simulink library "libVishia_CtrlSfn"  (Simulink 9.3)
settings: Solver=VariableStepAuto  StartTime=0.0  StopTime=10.0  RelTol=1e-3
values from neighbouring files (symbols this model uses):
  Tinit = 0.001    [TestOrthOsc_init.m]    (also in Test_PIDctrl_init.m)
  Tstep = 0.000050    (= 5e-05)    [TestOrthOsc_init.m]    (also in Test_PIDctrl_init.m = 0.0001)
undefined symbols (not defined in the file or in its folder): avgSteps, incrAvgSteps, P_WaveData_FB, P_WaveMng_FB, P_WaveMngIx_FB, src2genBus, stepA_WaveMngIx_FB, stepSimulink_AvgWave_FB, stepSimulink_WaveData_FB, stepSimulink_WaveMng_FB, u1, u2, void, work1, y1
libraries: lib_WaveMng x20, $bdroot x8, Lib_FunctionBlocks x4, lib_Conv x2

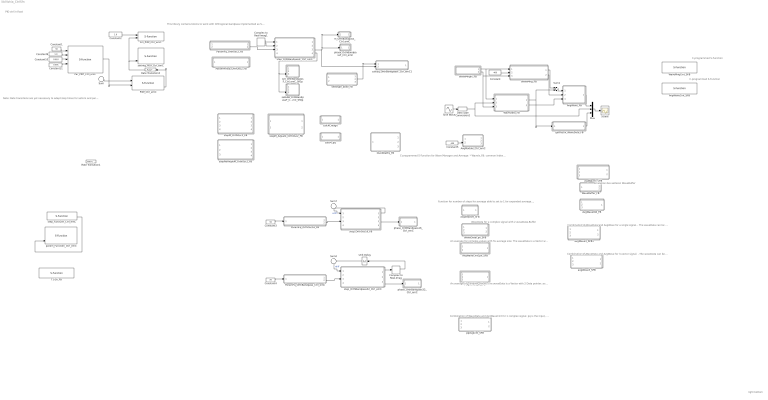
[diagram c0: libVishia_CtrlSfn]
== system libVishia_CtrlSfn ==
  note: Note: Rate transitions are yet necessary to adapt step times for setLim and param FBlock. The Limitation and parametrization may be occure in another step time. Note "step time" is the "sample time" in Simulink. "step" means more the control step.
  note: right bottom
  note: PID ctrl in float
  note: This library contains blocks to work with Orthogonal bandpass implemented as S-Function
  note: C-programmed S-Function
  note: C-programmed S-Function
  note: An average for complex values. The waveData is a Vector with 2 Data pointer. avg is a complex output.
  note: Function for number of steps for average able to set to 1 for expanded average. Parameter avgSteps
  note: C-programmed S-Function for Wave Manager and Average: * WaveIx_FB: common Index for one Buffer size. * WaveMng_FB: common manager for one average period but maybe more as one signal for averaging. * WaveData_FB; Buffer for data, for one signal value, but maybe for more as one average * AvgWave_FB: average for one signal and period. The connections ..._FB are references (ObjectOriented). The connections step... are only used to determine the calculation order.
  note: Combination of WaveData and AvgWaveCint for 1 complex signal. pq is the input, avg is the output. The waveData can be used for other accesses. It is a vector o2 2 pointer.
  note: An average for complex values with fix average size. The waveData is a Vector with 2 Data pointer. avg is a complex output.
  note: WaveData for a complex signal with 2 waveData-Buffer
  note: Emulation des aelteren WaveBuffer
  note: Combination of WaveData and AvgWave for a single signal. . The waveData can be used for other accesses. It is a pointer.
  note: Combination of WaveData and AvgWave for 3-vector signal. . The waveData can be used for other accesses. It is a vector o2 3 pointer.
  AvgModule_Ctrl_emC : Subsystem
  AvgWaveCintCpx_SFB : Subsystem
  AvgWaveCint_SFB : S-Function  LoadFcn=defWaveMngPtr  FunctionName=AvgWaveCint_SFB  SFunctionDeploymentMode=off  EnableBusSupport=off
  AvgWaveCpx_SFB : Subsystem
  AvgWaveOld_FB : Subsystem
  AvgWave_FB : Subsystem
  Complex to Real-Imag : ComplexToRealImag
  Complex to Real-Imag1 : ComplexToRealImag
  Constant : Constant  Value=400  OutDataTypeStr=single
  Constant1 : Constant  Value=50  OutDataTypeStr=single  SampleTime=-1
  Constant10 : Constant  Value=0.010  OutDataTypeStr=single  SampleTime=-1
  Constant11 : Constant  Value=0.001  OutDataTypeStr=single  SampleTime=-1
  Constant2 : Constant  Value=1.0  OutDataTypeStr=single  SampleTime=-1
  Constant3 : Constant  Value=50  OutDataTypeStr=single
  Constant4 : Constant  Value=50  OutDataTypeStr=single
  Constant5 : Constant  Value=400  OutDataTypeStr=single
  Constant9 : Constant  Value=1.0  OutDataTypeStr=single  SampleTime=-1
  Data Type Conversion2 : DataTypeConversion  OutDataTypeStr=single
  Mux : Mux  Inputs=3
  OscillDetFq_FB : Subsystem
  PIDf_Ctrl_emC : S-Function  FunctionName=step_PIDf_Ctrl_emC_SfH  Parameters=Tstep  SFunctionDeploymentMode=off  EnableBusSupport=off
  Par_PIDf_Ctrl_emC : S-Function  FunctionName=set_Par_PIDf_Ctrl_emC_SfH  Parameters=Tctrl yMax openLoop Tparam  SFunctionDeploymentMode=off  EnableBusSupport=off
  ParamFq_OrthBandpass_Ctrl_emC : Subsystem
  ParamFq_OrthOsc16_FB : Subsystem
  ParamFq_OrthOsc2_FB : Subsystem
  ParamPeriod_OrthOsc2_FB : Subsystem
  Rate Transition1 : RateTransition  OutPortSampleTimeOpt=Inherit  OutPortSampleTime=Tinit
  Rate Transition3 : RateTransition  OutPortSampleTimeOpt=Inherit  OutPortSampleTime=1.0
  Scope : Scope
  Sine Wave : Sin  Amplitude=4  Frequency=10.02*pi  SampleTime=Tstep
  Sum : Sum  Inputs=|+-
  Sum1 : Sum
  Sum2 : Sum  Inputs=+|-
  Sum7 : Sum  Inputs=+|-
  T1i16_FB : S-Function  FunctionName=stepY_T1i_Ctrl_emC_SfH  Parameters=Ts Tstep  SFunctionDeploymentMode=off  EnableBusSupport=off
  Unit Delay : UnitDelay  SampleTime=-1  HasFrameUpgradeWarning=on
  WaveBuffer_FB : Subsystem
  WaveDataCpx_SFB : Subsystem
  WaveData_FB : Subsystem
  WaveMngCint_SFB : S-Function  FunctionName=WaveMngCint_SFB  SFunctionDeploymentMode=off  EnableBusSupport=off
  WaveMngIx_FB : Subsystem
  WaveMng_FB : Subsystem
  avgStepSet_SFB : Subsystem
  avgWave3_CFB : Subsystem
  avgWave3_SFB : Subsystem
  avgWave3_SFB1 : Subsystem
  calcM_magn : Subsystem  TreatAsAtomicUnit=on
  calcM_pq : Subsystem  TreatAsAtomicUnit=on
  calcdq_OrthBandpassF_Ctrl_emC1 : Subsystem
  getPastIx_WaveData_FB : Subsystem
  lim_PIDf_Ctrl_emC : S-Function  FunctionName=setLim_PIDf_Ctrl_emC_SfOp  SFunctionDeploymentMode=off  EnableBusSupport=off
  m_OrthBandpass_Ctrl_emC : Subsystem
  param_FuncGen_Ctrl_emC : S-Function  FunctionName=param_FuncGen_Ctrl_emC_SfOp  SFunctionDeploymentMode=off  EnableBusSupport=off
  phase_OrthBandpass16_Ctrl_emC : Subsystem
  phase_OrthBandpass32_Ctrl_emC : Subsystem
  phase_OrthBandpassF_Ctrl_emC : Subsystem
  pqAvgCint_SFB : Subsystem
  setAngle_abwf_FB : Subsystem
  setIntg_PIDf_Ctrl_emC : S-Function  FunctionName=setIntg_PIDf_Ctrl_emC_SfOp  SFunctionDeploymentMode=off  EnableBusSupport=off
  set_OrthBandpassF_Ctrl_emC_SfOp : Subsystem
  setkAB_OrthBandpassF_Ctrl_emC_SfOp : Subsystem
  stepM_Adjustk_OrthOsc2_FB : Subsystem  TreatAsAtomicUnit=on
  stepM_OrthOsc2_FB : Subsystem  TreatAsAtomicUnit=on
  stepNoAngleM_OrthOsc2_FB : Subsystem  TreatAsAtomicUnit=on
  step_FuncGen_Ctrl_emC : S-Function  FunctionName=step_FuncGen_Ctrl_emC_SfH  Parameters=Tstep  SFunctionDeploymentMode=off  EnableBusSupport=off
  step_OrthBandpass32_Ctrl_emC : Subsystem
  step_OrthBandpassF_Ctrl_emC : Subsystem  LoadFcn=src2genBus.lib_OrthOsc_genBus();
  step_OrthOsc16_FB : Subsystem
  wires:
  Sum/1 -> PIDf_Ctrl_emC/1
  ? -> Sum/1  "w"
  ? -> Sum/2  "x"
  PIDf_Ctrl_emC/3 -> Rate Transition3/1
  Sum1/1 -> AvgWave_FB/1(In1)
  Data Type Conversion2/1 -> WaveData_FB/2(In3), Mux/2
  WaveMngIx_FB/2(Out1) -> WaveMng_FB/3(In2), WaveData_FB/3(In2)
  Constant/1 -> WaveMng_FB/2(In3)
  Sine Wave/1 -> Data Type Conversion2/1
  WaveData_FB/1(Out2) -> getPastIx_WaveData_FB/1(In2), Sum1/2
  WaveMng_FB/1(Out2) -> Sum1/1
  getPastIx_WaveData_FB/1(Out2) -> Mux/3
  WaveMng_FB/2(Out1) -> AvgWave_FB/2(In2)
  Mux/1 -> Scope/1
  WaveMngIx_FB/1(Out2) -> WaveData_FB/1(In1), WaveMng_FB/1(In1)
  WaveData_FB/2(Out1) -> AvgWave_FB/3(In4)
  AvgWave_FB/1(Out2) -> Mux/1
  Constant1/1 -> Par_PIDf_Ctrl_emC/1
  Constant10/1 -> Par_PIDf_Ctrl_emC/3
  Constant9/1 -> Par_PIDf_Ctrl_emC/2
  Constant11/1 -> Par_PIDf_Ctrl_emC/4
  Constant2/1 -> lim_PIDf_Ctrl_emC/1
  Par_PIDf_Ctrl_emC/1 -> PIDf_Ctrl_emC/2
  Rate Transition3/1 -> lim_PIDf_Ctrl_emC/2, setIntg_PIDf_Ctrl_emC/4
  ParamFq_OrthOsc16_FB/2(Out2) -> step_OrthOsc16_FB/3(In1)
  Sum7/1 -> step_OrthOsc16_FB/1(In4)  "xdiff"
  step_OrthOsc16_FB/1(Out3) -> Sum7/2
  ? -> Sum7/1
  Constant3/1 -> ParamFq_OrthOsc16_FB/1(In1)
  ? -> ?
  step_FuncGen_Ctrl_emC/2 -> param_FuncGen_Ctrl_emC/4
  ParamFq_OrthBandpass_Ctrl_emC/2(Out2) -> step_OrthBandpass32_Ctrl_emC/3(In1)
  Constant4/1 -> ParamFq_OrthBandpass_Ctrl_emC/1(In1)
  Sum2/1 -> step_OrthBandpass32_Ctrl_emC/1(In4)  "xdiff"
  Complex to Real-Imag/1 -> Unit Delay/1
  ? -> Sum2/1
  step_OrthBandpass32_Ctrl_emC/1(Out4) -> Complex to Real-Imag/1
  Unit Delay/1 -> Sum2/2
  Constant5/1 -> AvgModule_Ctrl_emC/2(In3)
  step_OrthBandpass32_Ctrl_emC/3(Out1) -> phase_OrthBandpass32_Ctrl_emC/1(In1)
  Complex to Real-Imag1/1 -> step_OrthBandpassF_Ctrl_emC/1(In4)
  Complex to Real-Imag1/2 -> step_OrthBandpassF_Ctrl_emC/2(In5)
  ParamFq_OrthOsc2_FB/2(Out2) -> step_OrthBandpassF_Ctrl_emC/3(In1)
  step_OrthBandpassF_Ctrl_emC/3(thiz_OrthOsc2_FB1) -> phase_OrthBandpassF_Ctrl_emC/1(In3), m_OrthBandpass_Ctrl_emC/1(In3), calcdq_OrthBandpassF_Ctrl_emC1/2(In3)
  step_OrthBandpassF_Ctrl_emC/4(thiz_OrthOsc2_FB) -> setkAB_OrthBandpassF_Ctrl_emC_SfOp/3(In3), set_OrthBandpassF_Ctrl_emC_SfOp/3(In3)
  setAngle_abwf_FB/2(thiz_Angle_abwmf_FB2) -> calcdq_OrthBandpassF_Ctrl_emC1/1(In1)
  step_OrthOsc16_FB/3(Out2) -> phase_OrthBandpass16_Ctrl_emC/1(In1)

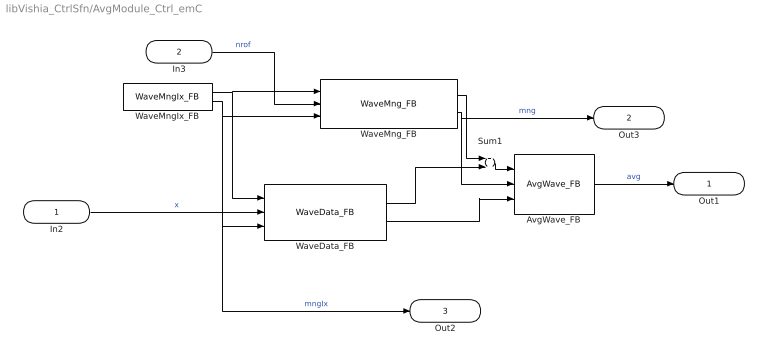
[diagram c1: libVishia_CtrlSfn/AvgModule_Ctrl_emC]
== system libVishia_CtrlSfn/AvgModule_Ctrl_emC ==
  In2 : Inport  OutDataTypeStr=single  PortDimensions=1
  In3 : Inport  Port=2  OutDataTypeStr=single  PortDimensions=1
  AvgWave_FB : $bdroot/AvgWave_FB  identObj=1
  Sum1 : Sum
  WaveData_FB : $bdroot/WaveData_FB  identObj=1  size=1024
  WaveMngIx_FB : $bdroot/WaveMngIx_FB  identObj=1  size=1024  Tstep=Tstep
  WaveMng_FB : $bdroot/WaveMng_FB  identObj=1
  Out1 : Outport  OutDataTypeStr=single  PortDimensions=1
  Out3 : Outport  Port=2  OutDataTypeStr=uint32  PortDimensions=1
  Out2 : Outport  Port=3  OutDataTypeStr=uint32  PortDimensions=1
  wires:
  WaveData_FB/1 -> Sum1/2
  WaveData_FB/2 -> AvgWave_FB/3
  WaveMngIx_FB/1 -> WaveData_FB/1, WaveMng_FB/1
  In3/1 -> WaveMng_FB/2  "nrof"
  In2/1 -> WaveData_FB/2  "x"
  WaveMng_FB/2 -> AvgWave_FB/2, Out3/1  "mng"
  Sum1/1 -> AvgWave_FB/1
  WaveMng_FB/1 -> Sum1/1
  WaveMngIx_FB/2 -> WaveMng_FB/3, Out2/1, WaveData_FB/3  "mngIx"
  AvgWave_FB/1 -> Out1/1  "avg"

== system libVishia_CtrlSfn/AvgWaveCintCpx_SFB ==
  In1 : Inport
  In5 : Inport  Port=2  OutDataTypeStr=P_WaveData_FB  PortDimensions=2
  AvgWaveCint_SFB : lib_WaveMng/AvgWaveCint_SFB  SFunctionSpec=stepSimulink_AvgWave_FB(void* work1, P_WaveMng_FB u1, P_WaveData_FB u2, single y1[1])  ShowSpec=off
  AvgWaveCint_SFB1 : lib_WaveMng/AvgWaveCint_SFB  SFunctionSpec=stepSimulink_AvgWave_FB(void* work1, P_WaveMng_FB u1, P_WaveData_FB u2, single y1[1])  ShowSpec=off
  Demux : Demux  Outputs=2
  Real-Imag to Complex2 : RealImagToComplex
  Out2 : Outport
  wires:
  In1/1 -> AvgWaveCint_SFB1/1, AvgWaveCint_SFB/1  "waveMngCiint"
  AvgWaveCint_SFB1/1 -> Real-Imag to Complex2/2
  Demux/1 -> AvgWaveCint_SFB/2  "waveD_xUApq[0]"
  AvgWaveCint_SFB/1 -> Real-Imag to Complex2/1
  In5/1 -> Demux/1  "waveData"
  Real-Imag to Complex2/1 -> Out2/1  "avg"
  Demux/2 -> AvgWaveCint_SFB1/2  "waveD_xUApq[1]"

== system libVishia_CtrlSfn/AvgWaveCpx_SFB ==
  In2 : Inport
  In1 : Inport  Port=2  OutDataTypeStr=uint32
  In5 : Inport  Port=3  OutDataTypeStr=uint32  PortDimensions=2
  AvgWave_FB : $bdroot/AvgWave_FB  identObj=0
  AvgWave_FB1 : $bdroot/AvgWave_FB  identObj=0
  Demux : Demux  Outputs=2
  Real-Imag to Complex2 : RealImagToComplex
  Out2 : Outport  OutDataTypeStr=single
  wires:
  Demux/2 -> AvgWave_FB1/3  "waveD_xUApq[1]"
  Real-Imag to Complex2/1 -> Out2/1  "avg"
  In5/1 -> Demux/1  "waveData"
  AvgWave_FB/1 -> Real-Imag to Complex2/1
  Demux/1 -> AvgWave_FB/3  "waveD_xUApq[0]"
  AvgWave_FB1/1 -> Real-Imag to Complex2/2
  In1/1 -> AvgWave_FB1/2, AvgWave_FB/2  "waveMng"
  In2/1 -> AvgWave_FB1/1, AvgWave_FB/1  "step"

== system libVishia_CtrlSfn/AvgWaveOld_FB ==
  In6 : Inport  OutDataTypeStr=P_WaveMngIx_FB
  In2 : Inport  Port=2  OutDataTypeStr=P_WaveData_FB
  In1 : Inport  Port=3  OutDataTypeStr=P_WaveMngIx_FB  PortDimensions=1
  AvgWave_SFB : lib_WaveMng/AvgWave_SFB  SFunctionSpec=stepSimulink_AvgWave_FB(void* work1, P_WaveMng_FB u1, P_WaveData_FB u2, single y1[1])  ShowSpec=off
  WaveMng_SFB : lib_WaveMng/WaveMng_SFB  SFunctionSpec=stepSimulink_WaveMng_FB(void* work1, P_WaveMngIx_FB u1, single u2, P_WaveMng_FB y1[1])  ShowSpec=off
  Out1 : Outport  OutDataTypeStr=single
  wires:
  WaveMng_SFB/1 -> AvgWave_SFB/1
  In6/1 -> WaveMng_SFB/1  "waveIxP"
  In1/1 -> WaveMng_SFB/2  "N"
  In2/1 -> AvgWave_SFB/2  "waveDataP"
  AvgWave_SFB/1 -> Out1/1  "Y"

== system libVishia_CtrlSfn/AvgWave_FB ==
  In1 : Inport  OutDataTypeStr=uint32
  In2 : Inport  Port=2  OutDataTypeStr=uint32
  In4 : Inport  Port=3  OutDataTypeStr=uint32
  AvgWave_SFB : S-Function  LoadFcn=defWaveMngPtr  FunctionName=step_AvgWave_FB_SfH  Parameters=123  SFunctionDeploymentMode=off  EnableBusSupport=off
  Out2 : Outport  OutDataTypeStr=single
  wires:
  In4/1 -> AvgWave_SFB/3  "WaveData"
  In2/1 -> AvgWave_SFB/2  "WaveMng_FB"
  AvgWave_SFB/1 -> Out2/1  "avg"
  In1/1 -> AvgWave_SFB/1  "step"

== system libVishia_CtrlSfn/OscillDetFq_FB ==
  In1 : Inport  OutDataTypeStr=single  PortDimensions=1
  SFunc : S-Function  LoadFcn=src2genBus.lib_OrthOsc_genBus();  FunctionName=step_OscillDetFq_FB_SfH  Parameters=ident Tstep dxstart dxmin amplMin stepNom stepMax  SFunctionDeploymentMode=off  EnableBusSupport=off
  Out4 : Outport  OutDataTypeStr=uint32  SampleTime=Tinit
  Out1 : Outport  Port=2  OutDataTypeStr=uint32
  Out3 : Outport  Port=3  OutDataTypeStr=single
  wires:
  SFunc/2 -> Out1/1  "thiz"
  In1/1 -> SFunc/1  "X"
  SFunc/3 -> Out3/1  "nSteps"
  SFunc/1 -> Out4/1  "OscillDetFq_FB"

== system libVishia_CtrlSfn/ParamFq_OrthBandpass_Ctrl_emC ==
  In1 : Inport  OutDataTypeStr=single
  param1_myOrthOsc : S-Function  FunctionName=setFq_Param_OrthBandpass32_Ctrl_emC_SfH  Parameters=0 Tstep TstepOrth  SFunctionDeploymentMode=off  EnableBusSupport=off
  Out1 : Outport  OutDataTypeStr=uint32  SampleTime=Tstep
  Out2 : Outport  Port=2  OutDataTypeStr=uint32  SampleTime=Tinit
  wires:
  param1_myOrthOsc/1 -> Out1/1  "thiz"
  param1_myOrthOsc/2 -> Out2/1  "Param_OrthOsc32_Ctrl_emC"
  In1/1 -> param1_myOrthOsc/1  "fq"

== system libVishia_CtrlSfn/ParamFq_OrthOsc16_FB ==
  In1 : Inport  OutDataTypeStr=single
  param1_myOrthOsc : S-Function  FunctionName=setFq_Param_OrthBandpass16_Ctrl_emC_SfH  Parameters=identObj Tstep TstepOrth  SFunctionDeploymentMode=off  EnableBusSupport=off
  Out1 : Outport  OutDataTypeStr=uint32  SampleTime=Tstep
  Out2 : Outport  Port=2  OutDataTypeStr=uint32  SampleTime=Tinit
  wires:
  param1_myOrthOsc/1 -> Out1/1  "thiz"
  param1_myOrthOsc/2 -> Out2/1  "Param_OrthOsc16_CtrlemC"
  In1/1 -> param1_myOrthOsc/1  "fq"

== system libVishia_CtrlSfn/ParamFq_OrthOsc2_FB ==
  In1 : Inport  OutDataTypeStr=single
  In2 : Inport  Port=2  OutDataTypeStr=single
  Terminator : Terminator
  param1_myOrthOsc : S-Function  FunctionName=setFq_Param_OrthBandpassF_Ctrl_emC_SfH  Parameters=identObj Tstep TstepOrth m_nom  SFunctionDeploymentMode=off  EnableBusSupport=off
  Out1 : Outport  OutDataTypeStr=uint32  SampleTime=Tstep
  Out2 : Outport  Port=2  OutDataTypeStr=uint32  SampleTime=Tinit
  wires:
  In1/1 -> param1_myOrthOsc/1  "fq"
  param1_myOrthOsc/2 -> Out2/1  "Param_OrthBandpassF_Ctrl_emC"
  param1_myOrthOsc/1 -> Out1/1  "thiz"
  In2/1 -> Terminator/1  "_"

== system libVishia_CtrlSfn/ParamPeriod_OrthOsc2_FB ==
  In1 : Inport  OutDataTypeStr=single
  sfn : S-Function  FunctionName=setPeriod_Param_OrthOsc2_FB_SfH  Parameters=identObj Tstep TstepOrth m_nom  SFunctionDeploymentMode=off  EnableBusSupport=off
  Out2 : Outport  OutDataTypeStr=uint32
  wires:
  sfn/1 -> Out2/1  "Param_OrthOsc2_FB"
  In1/1 -> sfn/1  "nPeriod"

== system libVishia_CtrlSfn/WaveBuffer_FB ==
  In9 : Inport  OutDataTypeStr=single  PortDimensions=1
  WaveData_SFB : lib_WaveMng/WaveData_SFB  SFunctionSpec=stepSimulink_WaveData_FB(void* work1, P_WaveMngIx_FB u1, single u2, P_WaveData_FB y1[1])  ShowSpec=off
  WaveMngIx_SFB : lib_WaveMng/WaveMngIx_SFB  SFunctionSpec=stepA_WaveMngIx_FB(void* work1, P_WaveMngIx_FB y1[1])  SParameter1=1024  ShowSpec=off
  Out3 : Outport  OutDataTypeStr=P_WaveData_FB  PortDimensions=1
  Out1 : Outport  Port=2  OutDataTypeStr=P_WaveMngIx_FB  PortDimensions=1
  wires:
  WaveMngIx_SFB/1 -> Out1/1, WaveData_SFB/1  "waveIxP"
  In9/1 -> WaveData_SFB/2  "X"
  WaveData_SFB/1 -> Out3/1  "WaveData"

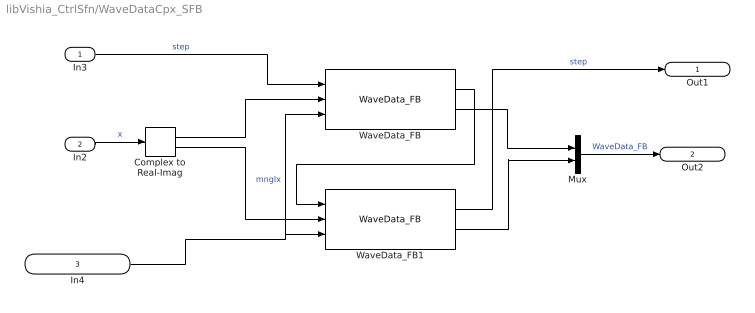
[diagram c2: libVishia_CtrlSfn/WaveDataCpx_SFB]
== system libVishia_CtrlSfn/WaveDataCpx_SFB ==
  In3 : Inport  OutDataTypeStr=uint32
  In2 : Inport  Port=2  OutDataTypeStr=single
  In4 : Inport  Port=3  OutDataTypeStr=uint32  SampleTime=Tinit
  Complex to Real-Imag : ComplexToRealImag
  Mux : Mux  Inputs=2
  WaveData_FB : $bdroot/WaveData_FB  identObj=0  size=sizeData
  WaveData_FB1 : $bdroot/WaveData_FB  identObj=0  size=sizeData
  Out1 : Outport  OutDataTypeStr=uint32
  Out2 : Outport  Port=2  OutDataTypeStr=uint32  SampleTime=Tinit
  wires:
  Complex to Real-Imag/1 -> WaveData_FB/2
  Complex to Real-Imag/2 -> WaveData_FB1/2
  In2/1 -> Complex to Real-Imag/1  "x"
  In3/1 -> WaveData_FB/1  "step"
  WaveData_FB/1 -> WaveData_FB1/1
  In4/1 -> WaveData_FB/3, WaveData_FB1/3  "mngIx"
  WaveData_FB/2 -> Mux/1
  WaveData_FB1/2 -> Mux/2
  Mux/1 -> Out2/1  "WaveData_FB"
  WaveData_FB1/1 -> Out1/1  "step"

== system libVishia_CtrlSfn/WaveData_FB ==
  In1 : Inport  OutDataTypeStr=uint32
  In3 : Inport  Port=2  OutDataTypeStr=single
  In2 : Inport  Port=3  OutDataTypeStr=uint32
  WaveData_SFB : S-Function  FunctionName=step_WaveData_FB_SfH  Parameters=0 size  SFunctionDeploymentMode=off  EnableBusSupport=off
  Out2 : Outport  OutDataTypeStr=uint32
  Out1 : Outport  Port=2  OutDataTypeStr=uint32
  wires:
  In3/1 -> WaveData_SFB/2  "X"
  In2/1 -> WaveData_SFB/3  "mngIx"
  WaveData_SFB/2 -> Out1/1  "WaveData_FB"
  WaveData_SFB/1 -> Out2/1  "step"
  In1/1 -> WaveData_SFB/1  "step"

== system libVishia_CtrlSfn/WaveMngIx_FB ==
  WaveMngIx_FB : S-Function  FunctionName=step_WaveMngIx_FB_SfH  Parameters=identObj size Tstep  SFunctionDeploymentMode=off  EnableBusSupport=off
  Out2 : Outport  OutDataTypeStr=uint32
  Out1 : Outport  Port=2  OutDataTypeStr=uint32
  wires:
  WaveMngIx_FB/2 -> Out1/1  "WaveMngIx_FB"
  WaveMngIx_FB/1 -> Out2/1  "step"

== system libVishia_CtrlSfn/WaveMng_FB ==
  In1 : Inport  OutDataTypeStr=uint32
  In3 : Inport  Port=2  OutDataTypeStr=single
  In2 : Inport  Port=3  OutDataTypeStr=uint32
  WaveMng_FB : S-Function  FunctionName=step_WaveMng_FB_SfH  Parameters=identObj  SFunctionDeploymentMode=off  EnableBusSupport=off
  Out2 : Outport  OutDataTypeStr=uint32
  Out1 : Outport  Port=2  OutDataTypeStr=uint32
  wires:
  WaveMng_FB/2 -> Out1/1  "WaveMng_FB"
  In2/1 -> WaveMng_FB/3  "mngIx"
  In3/1 -> WaveMng_FB/2  "nrofValuesAvg"
  In1/1 -> WaveMng_FB/1  "step"
  WaveMng_FB/1 -> Out2/1  "step"

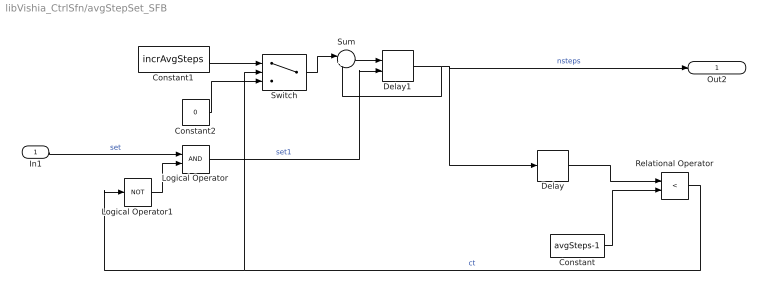
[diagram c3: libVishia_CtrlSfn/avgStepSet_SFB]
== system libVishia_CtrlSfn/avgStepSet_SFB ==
  In1 : Inport
  Constant : Constant  Value=avgSteps-1  OutDataTypeStr=single
  Constant1 : Constant  Value=incrAvgSteps  OutDataTypeStr=single
  Constant2 : Constant  Value=0  OutDataTypeStr=single
  Delay : Delay  DelayLength=1
  Delay1 : Delay  DelayLength=1  InitialCondition=1.0  ExternalReset=Level
  Logical Operator : Logic  AllPortsSameDT=off  OutDataTypeStr=boolean
  Logical Operator1 : Logic  Operator=NOT  AllPortsSameDT=off  OutDataTypeStr=boolean
  Relational Operator : RelationalOperator  Operator=<  OutDataTypeStr=boolean
  Sum : Sum  Inputs=|++
  Switch : Switch  Criteria=u2 ~= 0
  Out2 : Outport  OutDataTypeStr=single
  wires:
  Delay1/1 -> Delay/1, Out2/1, Sum/2  "nsteps"
  Constant/1 -> Relational Operator/2
  Delay/1 -> Relational Operator/1
  Sum/1 -> Delay1/1
  Constant1/1 -> Switch/1
  Logical Operator/1 -> Delay1/2  "set1"
  Switch/1 -> Sum/1
  Constant2/1 -> Switch/3
  Relational Operator/1 -> Logical Operator1/1, Switch/2  "ct"
  In1/1 -> Logical Operator/1  "set"
  Logical Operator1/1 -> Logical Operator/2

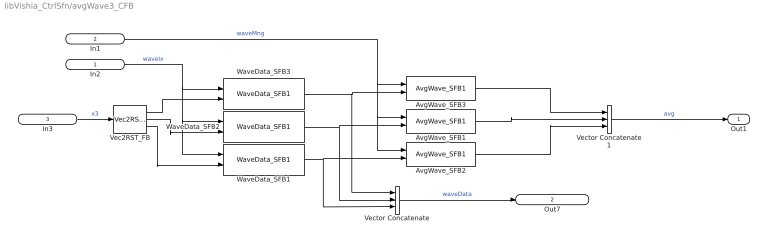
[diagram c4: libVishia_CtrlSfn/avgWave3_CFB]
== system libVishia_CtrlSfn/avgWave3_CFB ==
  In2 : Inport  OutDataTypeStr=Bus: WaveMngIx_FB
  In1 : Inport  Port=2  OutDataTypeStr=Bus: WaveMng_FB
  In3 : Inport  Port=3  OutDataTypeStr=single  PortDimensions=3
  AvgWave_SFB1 : lib_WaveMng/AvgWave_SFB1  SFunctionSpec=stepSimulink_AvgWave_FB(void* work1, P_WaveMng_FB u1, P_WaveData_FB u2, single y1[1])  ShowSpec=off
  AvgWave_SFB2 : lib_WaveMng/AvgWave_SFB1  SFunctionSpec=stepSimulink_AvgWave_FB(void* work1, P_WaveMng_FB u1, P_WaveData_FB u2, single y1[1])  ShowSpec=off
  AvgWave_SFB3 : lib_WaveMng/AvgWave_SFB1  SFunctionSpec=stepSimulink_AvgWave_FB(void* work1, P_WaveMng_FB u1, P_WaveData_FB u2, single y1[1])  ShowSpec=off
  Vec2RST_FB : lib_Conv/Vec2RST_FB
  Vector Concatenate : Concatenate  NumInputs=3
  Vector Concatenate1 : Concatenate  NumInputs=3
  WaveData_SFB1 : lib_WaveMng/WaveData_SFB1  SFunctionSpec=stepSimulink_WaveData_FB(void* work1, P_WaveMngIx_FB u1, single u2, P_WaveData_FB y1[1])  ShowSpec=off
  WaveData_SFB2 : lib_WaveMng/WaveData_SFB1  SFunctionSpec=stepSimulink_WaveData_FB(void* work1, P_WaveMngIx_FB u1, single u2, P_WaveData_FB y1[1])  ShowSpec=off
  WaveData_SFB3 : lib_WaveMng/WaveData_SFB1  SFunctionSpec=stepSimulink_WaveData_FB(void* work1, P_WaveMngIx_FB u1, single u2, P_WaveData_FB y1[1])  ShowSpec=off
  Out1 : Outport  OutDataTypeStr=single  PortDimensions=3
  Out7 : Outport  Port=2  OutDataTypeStr=Bus: WaveData_FB  PortDimensions=3
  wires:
  AvgWave_SFB2/1 -> Vector Concatenate1/3
  WaveData_SFB1/1 -> AvgWave_SFB2/2, Vector Concatenate/3
  Vec2RST_FB/3 -> WaveData_SFB1/2
  AvgWave_SFB1/1 -> Vector Concatenate1/2
  AvgWave_SFB3/1 -> Vector Concatenate1/1
  Vec2RST_FB/2 -> WaveData_SFB2/2
  WaveData_SFB2/1 -> AvgWave_SFB1/2, Vector Concatenate/2
  In2/1 -> WaveData_SFB3/1, WaveData_SFB1/1, WaveData_SFB2/1  "waveIx"
  WaveData_SFB3/1 -> AvgWave_SFB3/2, Vector Concatenate/1
  In1/1 -> AvgWave_SFB2/1, AvgWave_SFB1/1, AvgWave_SFB3/1  "waveMng"
  Vec2RST_FB/1 -> WaveData_SFB3/2
  Vector Concatenate1/1 -> Out1/1  "avg"
  In3/1 -> Vec2RST_FB/1  "x3"
  Vector Concatenate/1 -> Out7/1  "waveData"

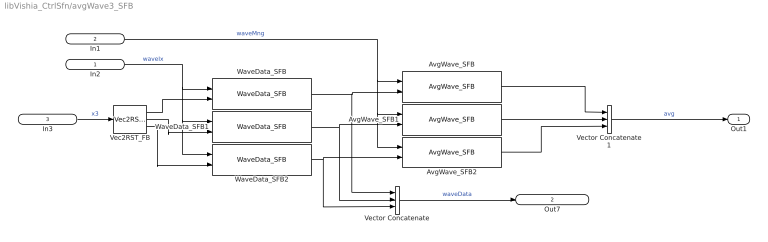
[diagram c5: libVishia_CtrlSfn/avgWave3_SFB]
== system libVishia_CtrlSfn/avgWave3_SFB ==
  In2 : Inport  OutDataTypeStr=P_WaveMngIx_FB
  In1 : Inport  Port=2  OutDataTypeStr=P_WaveMngCint_FB
  In3 : Inport  Port=3  OutDataTypeStr=single  PortDimensions=3
  AvgWave_SFB : lib_WaveMng/AvgWave_SFB  SFunctionSpec=stepSimulink_AvgWave_FB(void* work1, P_WaveMng_FB u1, P_WaveData_FB u2, single y1[1])  ShowSpec=off
  AvgWave_SFB1 : lib_WaveMng/AvgWave_SFB  SFunctionSpec=stepSimulink_AvgWave_FB(void* work1, P_WaveMng_FB u1, P_WaveData_FB u2, single y1[1])  ShowSpec=off
  AvgWave_SFB2 : lib_WaveMng/AvgWave_SFB  SFunctionSpec=stepSimulink_AvgWave_FB(void* work1, P_WaveMng_FB u1, P_WaveData_FB u2, single y1[1])  ShowSpec=off
  Vec2RST_FB : lib_Conv/Vec2RST_FB
  Vector Concatenate : Concatenate  NumInputs=3
  Vector Concatenate1 : Concatenate  NumInputs=3
  WaveData_SFB : lib_WaveMng/WaveData_SFB  SFunctionSpec=stepSimulink_WaveData_FB(void* work1, P_WaveMngIx_FB u1, single u2, P_WaveData_FB y1[1])  ShowSpec=off
  WaveData_SFB1 : lib_WaveMng/WaveData_SFB  SFunctionSpec=stepSimulink_WaveData_FB(void* work1, P_WaveMngIx_FB u1, single u2, P_WaveData_FB y1[1])  ShowSpec=off
  WaveData_SFB2 : lib_WaveMng/WaveData_SFB  SFunctionSpec=stepSimulink_WaveData_FB(void* work1, P_WaveMngIx_FB u1, single u2, P_WaveData_FB y1[1])  ShowSpec=off
  Out1 : Outport  OutDataTypeStr=single  PortDimensions=3
  Out7 : Outport  Port=2  OutDataTypeStr=P_WaveData_FB  PortDimensions=3
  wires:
  Vector Concatenate/1 -> Out7/1  "waveData"
  In3/1 -> Vec2RST_FB/1  "x3"
  Vector Concatenate1/1 -> Out1/1  "avg"
  Vec2RST_FB/1 -> WaveData_SFB/2
  In1/1 -> AvgWave_SFB/1, AvgWave_SFB2/1, AvgWave_SFB1/1  "waveMng"
  WaveData_SFB/1 -> Vector Concatenate/1, AvgWave_SFB/2
  In2/1 -> WaveData_SFB/1, WaveData_SFB2/1, WaveData_SFB1/1  "waveIx"
  WaveData_SFB1/1 -> Vector Concatenate/2, AvgWave_SFB1/2
  Vec2RST_FB/2 -> WaveData_SFB1/2
  AvgWave_SFB/1 -> Vector Concatenate1/1
  AvgWave_SFB1/1 -> Vector Concatenate1/2
  Vec2RST_FB/3 -> WaveData_SFB2/2
  WaveData_SFB2/1 -> Vector Concatenate/3, AvgWave_SFB2/2
  AvgWave_SFB2/1 -> Vector Concatenate1/3

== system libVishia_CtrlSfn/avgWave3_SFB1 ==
  In2 : Inport  OutDataTypeStr=P_WaveMngIx_FB
  In1 : Inport  Port=2  OutDataTypeStr=P_WaveMngCint_FB
  In3 : Inport  Port=3  OutDataTypeStr=single  PortDimensions=1
  AvgWave_SFB : lib_WaveMng/AvgWave_SFB  SFunctionSpec=stepSimulink_AvgWave_FB(void* work1, P_WaveMng_FB u1, P_WaveData_FB u2, single y1[1])  ShowSpec=off
  WaveData_SFB : lib_WaveMng/WaveData_SFB  SFunctionSpec=stepSimulink_WaveData_FB(void* work1, P_WaveMngIx_FB u1, single u2, P_WaveData_FB y1[1])  ShowSpec=off
  Out1 : Outport  OutDataTypeStr=single  PortDimensions=1
  Out7 : Outport  Port=2  OutDataTypeStr=P_WaveData_FB  PortDimensions=1
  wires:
  AvgWave_SFB/1 -> Out1/1
  In2/1 -> WaveData_SFB/1  "waveIx"
  In1/1 -> AvgWave_SFB/1  "waveMng"
  In3/1 -> WaveData_SFB/2  "x"
  WaveData_SFB/1 -> Out7/1, AvgWave_SFB/2  "waveData"

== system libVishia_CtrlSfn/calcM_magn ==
  In1 : Inport  OutDataTypeStr=uint32  Partition=on  PartitionDimension=1  PartitionWidth=1  PartitionOffset=0
  For Each : ForEach  DisableCoverage=on  IndexMode=One-based
  calcMagn_Orthi2_FB : S-Function  FunctionName=calcMagn_OrthOsc2_FB_SfOp  SFunctionDeploymentMode=off  EnableBusSupport=off
  Out3 : Outport  OutDataTypeStr=single  ConcatenationDimension=1
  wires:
  In1/1 -> calcMagn_Orthi2_FB/2  "thiz"
  calcMagn_Orthi2_FB/1 -> Out3/1  "ym"

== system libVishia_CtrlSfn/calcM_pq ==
  In1 : Inport  OutDataTypeStr=uint32  Partition=on  PartitionDimension=1  PartitionWidth=1  PartitionOffset=0
  For Each : ForEach  DisableCoverage=on  IndexMode=One-based
  step_Orthi2_FB : S-Function  FunctionName=calcpq_OrthOsc2_FB_SfOp  SFunctionDeploymentMode=off  EnableBusSupport=off
  Out3 : Outport  OutDataTypeStr=single  ConcatenationDimension=1
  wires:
  In1/1 -> step_Orthi2_FB/2  "thiz"
  step_Orthi2_FB/1 -> Out3/1  "ypq"

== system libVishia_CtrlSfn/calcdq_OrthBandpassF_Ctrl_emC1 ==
  In1 : Inport  OutDataTypeStr=uint32
  In3 : Inport  Port=2  OutDataTypeStr=uint32
  calcdq_OrthBandpassF_Ctrl_emC_SfOp : S-Function  FunctionName=calcpq_OrthBandpassF_Ctrl_emC_SfOp  SFunctionDeploymentMode=off  EnableBusSupport=off
  thiz_Angle_abwmf_FB : Outport  OutDataTypeStr=single
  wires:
  calcdq_OrthBandpassF_Ctrl_emC_SfOp/1 -> thiz_Angle_abwmf_FB/1  "dq"
  In3/1 -> calcdq_OrthBandpassF_Ctrl_emC_SfOp/2  "OrthBandpassF_Ctrl_emC"
  In1/1 -> calcdq_OrthBandpassF_Ctrl_emC_SfOp/1  "Angle_abwmf"

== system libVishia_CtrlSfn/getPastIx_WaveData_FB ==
  In2 : Inport  OutDataTypeStr=uint32
  getPastIx_WaveData_SFB : S-Function  FunctionName=getPastIx_WaveData_FB_SfH  Parameters=ixPast  SFunctionDeploymentMode=off  EnableBusSupport=off
  Out2 : Outport  OutDataTypeStr=single
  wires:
  In2/1 -> getPastIx_WaveData_SFB/1  "WaveData_FB"
  getPastIx_WaveData_SFB/1 -> Out2/1  "past"

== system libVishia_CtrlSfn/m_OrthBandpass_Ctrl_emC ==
  In3 : Inport  OutDataTypeStr=uint32
  calcMagn_OrthBandpassF_Ctrl_emC : S-Function  FunctionName=calcMagn_OrthBandpassF_Ctrl_emC_SfOp  SFunctionDeploymentMode=off  EnableBusSupport=off
  thiz_Angle_abwmf_FB : Outport  OutDataTypeStr=single
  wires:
  In3/1 -> calcMagn_OrthBandpassF_Ctrl_emC/1  "thiz"
  calcMagn_OrthBandpassF_Ctrl_emC/1 -> thiz_Angle_abwmf_FB/1  "m"

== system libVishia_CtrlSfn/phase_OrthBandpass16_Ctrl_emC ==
  In1 : Inport  OutDataTypeStr=uint32  PortDimensions=1
  phase_OrthBandpass32_Ctrl_emC : S-Function  FunctionName=phase_OrthBandpass16_Ctrl_emC_SfOp  SFunctionDeploymentMode=off  EnableBusSupport=off
  Out1 : Outport  OutDataTypeStr=int32  SampleTime=Tstep
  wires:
  phase_OrthBandpass32_Ctrl_emC/1 -> Out1/1  "phase"
  In1/1 -> phase_OrthBandpass32_Ctrl_emC/1  "thiz"

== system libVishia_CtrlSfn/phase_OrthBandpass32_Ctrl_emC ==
  In1 : Inport  OutDataTypeStr=uint32  PortDimensions=1
  phase_OrthBandpass32_Ctrl_emC : S-Function  FunctionName=phase_OrthBandpass32_Ctrl_emC_SfOp  SFunctionDeploymentMode=off  EnableBusSupport=off
  Out1 : Outport  OutDataTypeStr=int32  SampleTime=Tstep
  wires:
  In1/1 -> phase_OrthBandpass32_Ctrl_emC/1  "thiz"
  phase_OrthBandpass32_Ctrl_emC/1 -> Out1/1  "phase"

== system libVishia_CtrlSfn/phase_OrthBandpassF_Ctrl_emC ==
  In3 : Inport  OutDataTypeStr=uint32
  phase_OrthBandpassF_Ctrl_emC_SfOp : S-Function  FunctionName=phase_OrthBandpassF_Ctrl_emC_SfOp  SFunctionDeploymentMode=off  EnableBusSupport=off
  thiz_Angle_abwmf_FB : Outport  OutDataTypeStr=single
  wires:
  phase_OrthBandpassF_Ctrl_emC_SfOp/1 -> thiz_Angle_abwmf_FB/1  "ph"
  In3/1 -> phase_OrthBandpassF_Ctrl_emC_SfOp/1  "thiz"

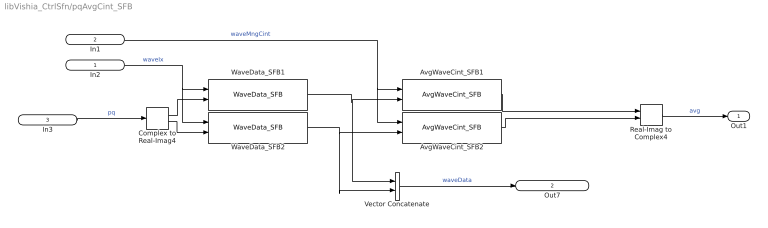
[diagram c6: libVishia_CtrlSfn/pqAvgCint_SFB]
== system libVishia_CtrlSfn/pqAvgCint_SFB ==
  In2 : Inport  OutDataTypeStr=P_WaveMngIx_FB
  In1 : Inport  Port=2  OutDataTypeStr=P_WaveMngCint_FB
  In3 : Inport  Port=3  OutDataTypeStr=single
  AvgWaveCint_SFB1 : Lib_FunctionBlocks/AvgWaveCint_SFB  SFunctionSpec=stepSimulink_AvgWave_FB(void* work1, P_WaveMng_FB u1, P_WaveData_FB u2, single y1[1])  ShowSpec=off
  AvgWaveCint_SFB2 : Lib_FunctionBlocks/AvgWaveCint_SFB  SFunctionSpec=stepSimulink_AvgWave_FB(void* work1, P_WaveMng_FB u1, P_WaveData_FB u2, single y1[1])  ShowSpec=off
  Complex to Real-Imag4 : ComplexToRealImag
  Real-Imag to Complex4 : RealImagToComplex
  Vector Concatenate : Concatenate
  WaveData_SFB1 : Lib_FunctionBlocks/WaveData_SFB  SFunctionSpec=stepSimulink_WaveData_FB(void* work1, P_WaveMngIx_FB u1, single u2, P_WaveData_FB y1[1])  ShowSpec=off
  WaveData_SFB2 : Lib_FunctionBlocks/WaveData_SFB  SFunctionSpec=stepSimulink_WaveData_FB(void* work1, P_WaveMngIx_FB u1, single u2, P_WaveData_FB y1[1])  ShowSpec=off
  Out1 : Outport  OutDataTypeStr=single
  Out7 : Outport  Port=2  OutDataTypeStr=P_WaveData_FB  PortDimensions=2
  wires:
  AvgWaveCint_SFB2/1 -> Real-Imag to Complex4/2
  AvgWaveCint_SFB1/1 -> Real-Imag to Complex4/1
  Complex to Real-Imag4/2 -> WaveData_SFB2/2
  WaveData_SFB2/1 -> Vector Concatenate/2, AvgWaveCint_SFB2/2
  In2/1 -> WaveData_SFB2/1, WaveData_SFB1/1  "waveIx"
  WaveData_SFB1/1 -> Vector Concatenate/1, AvgWaveCint_SFB1/2
  In1/1 -> AvgWaveCint_SFB2/1, AvgWaveCint_SFB1/1  "waveMngCint"
  Complex to Real-Imag4/1 -> WaveData_SFB1/2
  Real-Imag to Complex4/1 -> Out1/1  "avg"
  In3/1 -> Complex to Real-Imag4/1  "pq"
  Vector Concatenate/1 -> Out7/1  "waveData"

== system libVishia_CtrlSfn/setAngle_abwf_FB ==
  In3 : Inport  OutDataTypeStr=int32
  In2 : Inport  Port=2  OutDataTypeStr=single
  mAngle : Constant  OutDataTypeStr=single
  set_Angle_abwmf_FB : S-Function  FunctionName=set_Angle_abwmf_FB_SfH  Parameters=identObj Tstep  SFunctionDeploymentMode=off  EnableBusSupport=off
  thiz_Angle_abwmf_FB1 : Outport  OutDataTypeStr=single
  thiz_Angle_abwmf_FB2 : Outport  Port=2  OutDataTypeStr=uint32  SampleTime=Tstep
  thiz_Angle_abwmf_FB : Outport  Port=3  OutDataTypeStr=uint32  SampleTime=Tinit
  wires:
  In3/1 -> set_Angle_abwmf_FB/1  "gi"
  In2/1 -> set_Angle_abwmf_FB/2  "fq"
  mAngle/1 -> set_Angle_abwmf_FB/3
  set_Angle_abwmf_FB/1 -> thiz_Angle_abwmf_FB1/1  "rad"
  set_Angle_abwmf_FB/3 -> thiz_Angle_abwmf_FB/1  "Angle_abgm_FB"
  set_Angle_abwmf_FB/2 -> thiz_Angle_abwmf_FB2/1  "thiz"

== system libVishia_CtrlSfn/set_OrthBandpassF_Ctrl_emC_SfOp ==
  In4 : Inport  OutDataTypeStr=boolean
  In1 : Inport  Port=2  OutDataTypeStr=single
  In3 : Inport  Port=3  OutDataTypeStr=uint32
  Complex to Real-Imag : ComplexToRealImag
  set_OrthBandpassF_Ctrl_emC_SfOp : S-Function  FunctionName=set_OrthBandpassF_Ctrl_emC_SfOp  SFunctionDeploymentMode=off  EnableBusSupport=off
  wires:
  In1/1 -> Complex to Real-Imag/1  "ab"
  In3/1 -> set_OrthBandpassF_Ctrl_emC_SfOp/4  "thizi"
  Complex to Real-Imag/2 -> set_OrthBandpassF_Ctrl_emC_SfOp/3  "b"
  In4/1 -> set_OrthBandpassF_Ctrl_emC_SfOp/1  "set"
  Complex to Real-Imag/1 -> set_OrthBandpassF_Ctrl_emC_SfOp/2

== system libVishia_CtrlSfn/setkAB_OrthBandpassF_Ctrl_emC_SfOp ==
  In1 : Inport  OutDataTypeStr=single
  In2 : Inport  Port=2  OutDataTypeStr=single
  In3 : Inport  Port=3  OutDataTypeStr=uint32
  setkAB_OrthBandpassF_Ctrl_emC_SfOp : S-Function  FunctionName=setkAB_OrthBandpassF_Ctrl_emC_SfOp  SFunctionDeploymentMode=off  EnableBusSupport=off
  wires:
  In2/1 -> setkAB_OrthBandpassF_Ctrl_emC_SfOp/2  "kB"
  In3/1 -> setkAB_OrthBandpassF_Ctrl_emC_SfOp/3  "thizi"
  In1/1 -> setkAB_OrthBandpassF_Ctrl_emC_SfOp/1  "kA"

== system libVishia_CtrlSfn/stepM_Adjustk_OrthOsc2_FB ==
  In1 : Inport  OutDataTypeStr=uint32  PortDimensions=1  Partition=on  PartitionDimension=1  PartitionWidth=1  PartitionOffset=0
  In4 : Inport  Port=2  OutDataTypeStr=single  Partition=on  PartitionDimension=1  PartitionWidth=1  PartitionOffset=0
  For Each : ForEach  DisableCoverage=on  IndexMode=One-based
  step_Orthi2_FB_SFunc : S-Function  LoadFcn=src2genBus.lib_OrthOsc_genBus();  FunctionName=step_Adjustk_OrthOsc2_FB_SfH  Parameters=ident max_e kHi kNormal Tstep Tdecay  SFunctionDeploymentMode=off  EnableBusSupport=off
  Out1 : Outport  OutDataTypeStr=uint32  ConcatenationDimension=1
  Out2 : Outport  Port=2  OutDataTypeStr=uint32  ConcatenationDimension=1
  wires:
  In4/1 -> step_Orthi2_FB_SFunc/2  "xdiff"
  In1/1 -> step_Orthi2_FB_SFunc/1  "orthOsc"
  step_Orthi2_FB_SFunc/1 -> Out1/1  "thiz"
  step_Orthi2_FB_SFunc/2 -> Out2/1  "Adjustk"

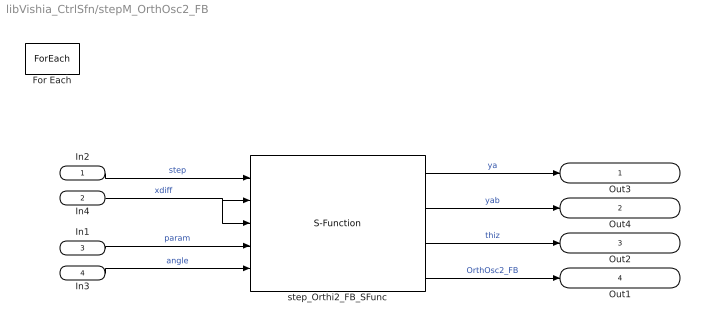
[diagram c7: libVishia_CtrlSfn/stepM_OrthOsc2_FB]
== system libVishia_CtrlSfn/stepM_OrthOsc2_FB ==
  In2 : Inport  OutDataTypeStr=uint32  PortDimensions=1
  In4 : Inport  Port=2  OutDataTypeStr=single  Partition=on  PartitionDimension=1  PartitionWidth=1  PartitionOffset=0
  In1 : Inport  Port=3  OutDataTypeStr=uint32  PortDimensions=1
  In3 : Inport  Port=4  OutDataTypeStr=uint32
  For Each : ForEach  DisableCoverage=on  IndexMode=One-based
  step_Orthi2_FB_SFunc : S-Function  LoadFcn=src2genBus.lib_OrthOsc_genBus();  FunctionName=step_OrthOsc2_FB_SfH  Parameters=kA kB ident Tstep  SFunctionDeploymentMode=off  EnableBusSupport=off
  Out3 : Outport  OutDataTypeStr=single  ConcatenationDimension=1
  Out4 : Outport  Port=2  OutDataTypeStr=single  ConcatenationDimension=1
  Out2 : Outport  Port=3  OutDataTypeStr=uint32  SampleTime=Tstep  ConcatenationDimension=1
  Out1 : Outport  Port=4  OutDataTypeStr=uint32  SampleTime=Tinit  ConcatenationDimension=1
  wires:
  In3/1 -> step_Orthi2_FB_SFunc/5  "angle"
  In1/1 -> step_Orthi2_FB_SFunc/4  "param"
  step_Orthi2_FB_SFunc/4 -> Out1/1  "OrthOsc2_FB"
  In4/1 -> step_Orthi2_FB_SFunc/2, step_Orthi2_FB_SFunc/3  "xdiff"
  step_Orthi2_FB_SFunc/1 -> Out3/1  "ya"
  step_Orthi2_FB_SFunc/2 -> Out4/1  "yab"
  step_Orthi2_FB_SFunc/3 -> Out2/1  "thiz"
  In2/1 -> step_Orthi2_FB_SFunc/1  "step"

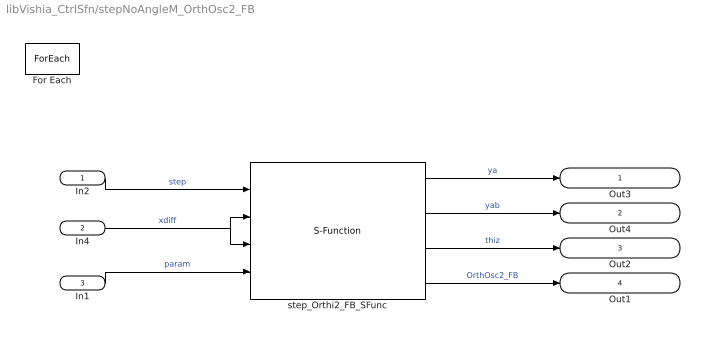
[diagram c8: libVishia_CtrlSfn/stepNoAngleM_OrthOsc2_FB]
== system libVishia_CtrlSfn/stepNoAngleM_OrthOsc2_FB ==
  In2 : Inport  OutDataTypeStr=uint32  PortDimensions=1
  In4 : Inport  Port=2  OutDataTypeStr=single  Partition=on  PartitionDimension=1  PartitionWidth=1  PartitionOffset=0
  In1 : Inport  Port=3  OutDataTypeStr=uint32  PortDimensions=1
  For Each : ForEach  DisableCoverage=on  IterateSubsysMaskParameter=off,off,off  IndexMode=One-based
  step_Orthi2_FB_SFunc : S-Function  LoadFcn=src2genBus.lib_OrthOsc_genBus();  FunctionName=stepNoAngle_OrthOsc2_FB_SfH  Parameters=kA kB ident Tstep  SFunctionDeploymentMode=off  EnableBusSupport=off
  Out3 : Outport  OutDataTypeStr=single  ConcatenationDimension=1
  Out4 : Outport  Port=2  OutDataTypeStr=single  ConcatenationDimension=1
  Out2 : Outport  Port=3  OutDataTypeStr=uint32  SampleTime=Tstep  ConcatenationDimension=1
  Out1 : Outport  Port=4  OutDataTypeStr=uint32  SampleTime=Tinit  ConcatenationDimension=1
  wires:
  step_Orthi2_FB_SFunc/2 -> Out4/1  "yab"
  step_Orthi2_FB_SFunc/1 -> Out3/1  "ya"
  In4/1 -> step_Orthi2_FB_SFunc/3, step_Orthi2_FB_SFunc/2  "xdiff"
  step_Orthi2_FB_SFunc/4 -> Out1/1  "OrthOsc2_FB"
  In1/1 -> step_Orthi2_FB_SFunc/4  "param"
  step_Orthi2_FB_SFunc/3 -> Out2/1  "thiz"
  In2/1 -> step_Orthi2_FB_SFunc/1  "step"

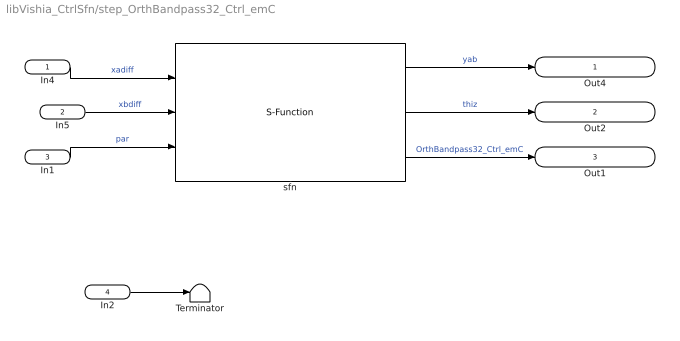
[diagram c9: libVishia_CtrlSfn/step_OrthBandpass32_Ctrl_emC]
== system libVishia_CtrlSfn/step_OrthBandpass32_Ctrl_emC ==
  In4 : Inport  OutDataTypeStr=int32
  In5 : Inport  Port=2  OutDataTypeStr=int32
  In1 : Inport  Port=3  OutDataTypeStr=uint32  PortDimensions=1
  In2 : Inport  Port=4  OutDataTypeStr=uint32  PortDimensions=1
  Terminator : Terminator
  sfn : S-Function  LoadFcn=src2genBus.lib_OrthOsc_genBus();  FunctionName=stepSmlk_OrthBandpass32_Ctrl_emC_SfH  Parameters=kA kB 0 Tstep  SFunctionDeploymentMode=off  EnableBusSupport=off
  Out4 : Outport  OutDataTypeStr=int32
  Out2 : Outport  Port=2  OutDataTypeStr=uint32
  Out1 : Outport  Port=3  OutDataTypeStr=uint32
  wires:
  sfn/3 -> Out1/1  "OrthBandpass32_Ctrl_emC"
  sfn/1 -> Out4/1  "yab"
  In1/1 -> sfn/3  "par"
  In4/1 -> sfn/1  "xadiff"
  sfn/2 -> Out2/1  "thiz"
  In5/1 -> sfn/2  "xbdiff"
  In2/1 -> Terminator/1  "."

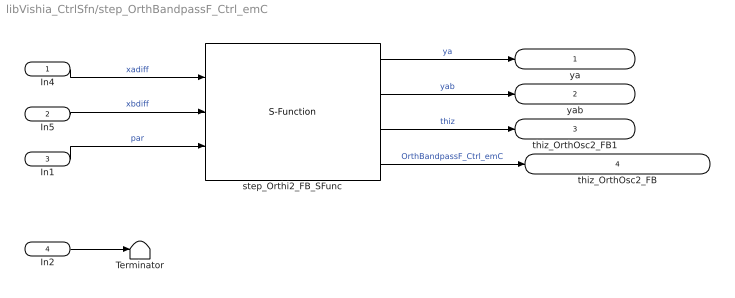
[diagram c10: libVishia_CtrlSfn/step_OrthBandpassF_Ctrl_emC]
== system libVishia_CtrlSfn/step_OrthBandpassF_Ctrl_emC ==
  In4 : Inport  OutDataTypeStr=single
  In5 : Inport  Port=2  OutDataTypeStr=single
  In1 : Inport  Port=3  OutDataTypeStr=uint32  PortDimensions=1
  In2 : Inport  Port=4  OutDataTypeStr=uint32  PortDimensions=1
  Terminator : Terminator
  step_Orthi2_FB_SFunc : S-Function  LoadFcn=src2genBus.lib_OrthOsc_genBus();  FunctionName=stepSmlk_OrthBandpassF_Ctrl_emC_SfH  Parameters=kA kB 0 Tstep  SFunctionDeploymentMode=off  EnableBusSupport=off
  ya : Outport  OutDataTypeStr=single
  yab : Outport  Port=2  OutDataTypeStr=single
  thiz_OrthOsc2_FB1 : Outport  Port=3  OutDataTypeStr=uint32
  thiz_OrthOsc2_FB : Outport  Port=4  OutDataTypeStr=uint32
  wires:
  step_Orthi2_FB_SFunc/4 -> thiz_OrthOsc2_FB/1  "OrthBandpassF_Ctrl_emC"
  In1/1 -> step_Orthi2_FB_SFunc/3  "par"
  In4/1 -> step_Orthi2_FB_SFunc/1  "xadiff"
  step_Orthi2_FB_SFunc/2 -> yab/1  "yab"
  step_Orthi2_FB_SFunc/1 -> ya/1  "ya"
  In5/1 -> step_Orthi2_FB_SFunc/2  "xbdiff"
  step_Orthi2_FB_SFunc/3 -> thiz_OrthOsc2_FB1/1  "thiz"
  In2/1 -> Terminator/1  "."

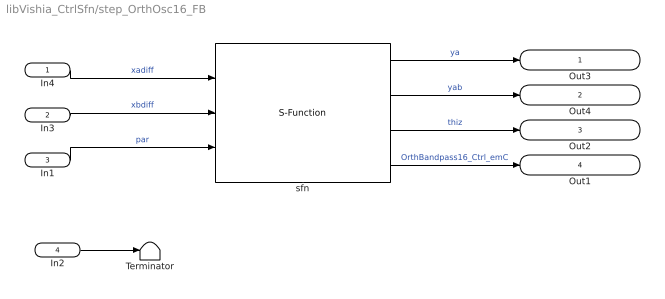
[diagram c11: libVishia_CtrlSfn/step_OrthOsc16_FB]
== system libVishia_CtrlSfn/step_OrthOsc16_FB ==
  In4 : Inport  OutDataTypeStr=int16
  In3 : Inport  Port=2  OutDataTypeStr=int16
  In1 : Inport  Port=3  OutDataTypeStr=uint32  PortDimensions=1
  In2 : Inport  Port=4  OutDataTypeStr=uint32  PortDimensions=1
  Terminator : Terminator
  sfn : S-Function  LoadFcn=src2genBus.lib_OrthOsc_genBus();  FunctionName=stepSmlk_OrthBandpass16_Ctrl_emC_SfH  Parameters=kA kB 0 Tstep  SFunctionDeploymentMode=off  EnableBusSupport=off
  Out3 : Outport  OutDataTypeStr=int16
  Out4 : Outport  Port=2  OutDataTypeStr=int16
  Out2 : Outport  Port=3  OutDataTypeStr=uint32
  Out1 : Outport  Port=4  OutDataTypeStr=uint32
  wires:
  sfn/4 -> Out1/1  "OrthBandpass16_Ctrl_emC"
  sfn/1 -> Out3/1  "ya"
  sfn/2 -> Out4/1  "yab"
  In1/1 -> sfn/3  "par"
  In4/1 -> sfn/1  "xadiff"
  sfn/3 -> Out2/1  "thiz"
  In3/1 -> sfn/2  "xbdiff"
  In2/1 -> Terminator/1  "."
